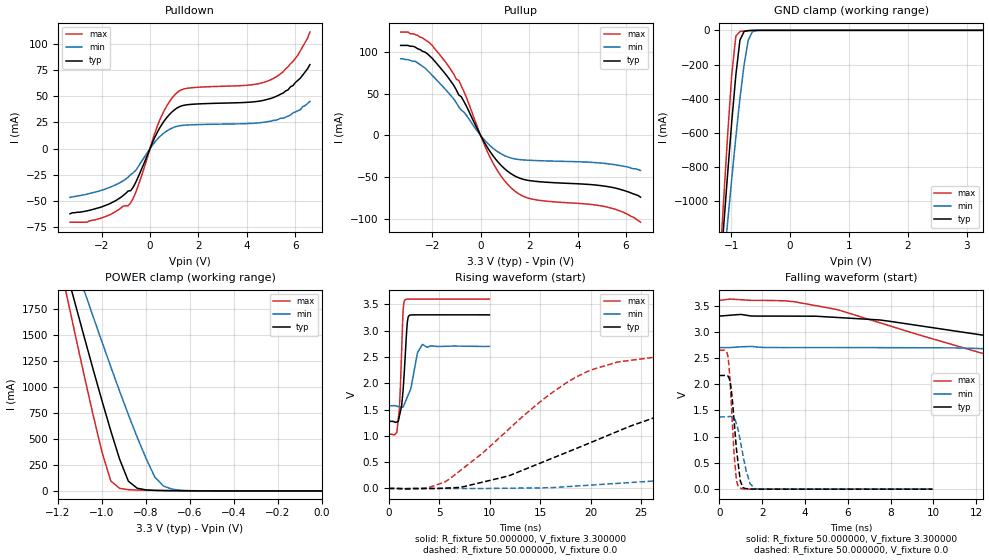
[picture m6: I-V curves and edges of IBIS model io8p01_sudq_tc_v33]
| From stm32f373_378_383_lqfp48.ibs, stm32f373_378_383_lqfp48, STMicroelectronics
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|   Model io8p01_sudq_tc_v33
[Model]  io8p01_sudq_tc_v33
Model_type I/O
Polarity   Non-Inverting
Enable   Active-Low
Vinl =   0.990000V
Vinh =   2.310000V
Vmeas =  1.650000V
Cref =   50.000000pF
Rref =   100.000000M
Vref =   0.0V
C_comp   1.325200pF   1.251200pF   1.426700pF
[Temperature Range]   25.000000   0.125000k   -40.000000
[Pullup Reference]   3.300000V   2.700000V   3.600000V
[Pulldown Reference]   0.0V   0.0V   0.0V
[POWER Clamp Reference]   3.300000V   2.700000V   3.600000V
[GND Clamp Reference]   0.0V   0.0V   0.0V
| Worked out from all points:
|   slope of the pulldown table from 0 to 0.495 V, typ, clamps not added: 21.3 ohm
|   slope of the pullup table from 0 to 0.495 V, typ, clamps not added: 20.9 ohm
|   GND clamp passes 1 mA (typ) near -0.67 V on its own axis
|   POWER clamp passes 1 mA (typ) near -0.60 V on its own axis
|   rising waveform, R_fixture 50.000000, V_fixture 3.300000: 20-80 % time 413ps typ, 774ps min, 302ps max; typ from 1.27 V to 3.3 V
|   rising waveform, R_fixture 50.000000, V_fixture 0.0: 20-80 % time 18.6ns typ, 46.7ns min, 10.2ns max; typ from 0 V to 2.17 V
|   falling waveform, R_fixture 50.000000, V_fixture 3.300000: 20-80 % time 26.2ns typ, 44.8ns min, 16.3ns max; typ from 3.3 V to 1.27 V
|   falling waveform, R_fixture 50.000000, V_fixture 0.0: 20-80 % time 299ps typ, 415ps min, 225ps max; typ from 2.17 V to 0 V
[Pulldown]
|Voltage   I(typ)   I(min)   I(max)
-3.3V     -62mA      -46.4mA    -70mA
-2V       -55.5mA    -39.6mA    -66mA
-800mV    -40.04mA   -24.89mA   -51.58mA
-500mV    -27.57mA   -17.6mA    -36.07mA
400mV     19.71mA    11.36mA    27.01mA
700mV     29.83mA    16.93mA    40.97mA
1.1V      38.46mA    21.2mA     53.02mA
1.6V      41.98mA    22.62mA    57.7mA
4.1V      44.26mA    24mA       60.59mA
5V        47.9mA     26.3mA     65.8mA
5.9V      60mA       34mA       83mA
6.6V      80mA       45mA       111mA
[Pullup]
|Voltage   I(typ)   I(min)   I(max)
-3.3V     108mA      92mA       124mA
-2.7V     106mA      89mA       121mA
-2.2V     98mA       78.2mA     113mA
-1.4V     71.8mA     53.5mA     86.1mA
-900mV    48.51mA    34.23mA    66.14mA
-700mV    41.33mA    28.36mA    53.31mA
400mV     -19.77mA   -12.52mA   -26.8mA
900mV     -37.48mA   -22.89mA   -50.99mA
1.4V      -48.39mA   -28.06mA   -66.43mA
2.2V      -54.79mA   -29.98mA   -76.75mA
5.3V      -61.6mA    -34.2mA    -86.4mA
6.6V      -74mA      -42mA      -104mA
[GND_clamp]
|Voltage   I(typ)   I(min)   I(max)
-3.3V     -9.739A    -9.975A    -9.587A
-1.2V     -1.489A    -1.65A     -1.416A
-1.13V    -1.162A    -1.385A    -1.009A
-1.06V    -842.2mA   -1.125A    -616.9mA
-990mV    -537.1mA   -870.1mA   -263mA
-920mV    -262.4mA   -625.3mA   -33.96mA
-850mV    -56.94mA   -397.4mA   -7.08mA
-780mV    -7.011mA   -202.2mA   -3.71mA
-710mV    -1.778mA   -58.23mA   -1.736mA
-640mV    -550uA     -8.783mA   -542.4uA
-570mV    -109.8uA   -1.292mA   -86.89uA
3.28V     0A         0A         0A
[POWER_clamp]
|Voltage   I(typ)   I(min)   I(max)
-3.28V    9.897A     9.838A     9.594A
-1.16V    2.103A     2.419A     1.88A
-1.12V    1.788A     2.17A      1.488A
-1.08V    1.476A     1.923A     1.102A
-1V       868.1mA    1.435A     373.1mA
-960mV    578.2mA    1.196A     96.06mA
-880mV    93.24mA    734.1mA    12.01mA
-840mV    26.3mA     517.4mA    8.56mA
-760mV    5.106mA    134mA      5.119mA
-720mV    3.355mA    46.34mA    3.808mA
-600mV    1.005mA    2.564mA    1.072mA
0V        0A         0A         0A
[Ramp]
| variable   typ   min   max
dV/dt_r  1.30032/18.57789n   0.82758/46.63597n   1.58898/10.20808n
dV/dt_f  1.21512/26.20754n   0.67770/44.52562n   1.54248/16.27144n
R_load = 50.000000
[Rising Waveform]
R_fixture= 50.000000
V_fixture= 3.300000
V_fixture_min= 2.700000
V_fixture_max= 3.600000
|time   V(typ)   V(min)   V(max)
0s        1.275V     1.571V     1.029V
820.8ps   1.264V     1.564V     1.094V
1.061ns   1.376V     1.551V     1.534V
1.281ns   1.568V     1.547V     2.601V
1.441ns   1.916V     1.552V     3.417V
1.602ns   2.401V     1.626V     3.581V
1.942ns   3.262V     1.783V     3.599V
2.843ns   3.3V       2.575V     3.6V
3.323ns   3.3V       2.736V     3.6V
9.97ns    3.3V       2.7V       3.6V
[Rising Waveform]
R_fixture= 50.000000
V_fixture= 0.0
V_fixture_min= 0.0
V_fixture_max= 0.0
|time   V(typ)   V(min)   V(max)
0s        1.051nV    9.611nV    1.582nV
5.506ns   6.079mV    -223.4uV   117mV
12.01ns   250mV      4.962mV    1.15V
19.52ns   835.6mV    57.91mV    2.209V
28.03ns   1.462V     163.7mV    2.536V
37.04ns   1.885V     351.1mV    2.61V
48.05ns   2.066V     584.2mV    2.634V
69.07ns   2.144V     972.6mV    2.648V
107.6ns   2.167V     1.295V     2.648V
249.2ns   2.167V     1.378V     2.648V
[Falling Waveform]
R_fixture= 50.000000
V_fixture= 3.300000
V_fixture_min= 2.700000
V_fixture_max= 3.600000
|time   V(typ)   V(min)   V(max)
0s        3.3V       2.7V       3.6V
3.003ns   3.3V       2.7V       3.593V
5.506ns   3.274V     2.7V       3.425V
14.01ns   2.833V     2.657V     2.387V
20.52ns   2.429V     2.57V      1.799V
28.53ns   2.037V     2.409V     1.344V
36.54ns   1.745V     2.248V     1.147V
60.06ns   1.365V     1.895V     1.043V
88.09ns   1.286V     1.682V     1.029V
249.2ns   1.275V     1.571V     1.029V
[Falling Waveform]
R_fixture= 50.000000
V_fixture= 0.0
V_fixture_min= 0.0
V_fixture_max= 0.0
|time   V(typ)   V(min)   V(max)
0s        2.167V     1.378V     2.648V
400.4ps   2.157V     1.382V     2.528V
540.5ps   1.954V     1.385V     1.776V
700.7ps   1.252V     1.342V     609.4mV
800.8ps   758mV      1.241V     166.2mV
940.9ps   287.5mV    1.008V     27.92mV
1.081ns   48.23mV    700.3mV    8.134mV
1.261ns   9.991mV    340.6mV    1.76mV
1.682ns   587.3uV    4.268mV    162.8uV
9.97ns    1.051nV    9.611nV    1.582nV
